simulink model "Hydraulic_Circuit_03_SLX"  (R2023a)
settings: Solver=ode23s  StartTime=0.0  StopTime=10.0  MaxStep=0.001  RelTol=1e-3
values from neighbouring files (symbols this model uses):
  C_5 = 0.001*m^3/Pa    (= 0.001)    [Hydraulic_Circuit_03_EQN.m]    (also in Hydraulic_Circuit_03_SLX_m.m; Electric_Circuit_02_EQN.m; Electric_Circuit_02_SLX_m.m; Electric_Circuit_04_EQN.m)
  C_8 = 0.001*m^3/Pa    (= 0.001)    [Hydraulic_Circuit_03_EQN.m]    (also in Hydraulic_Circuit_03_SLX_m.m; BIG_EC_Simscape_EQN.m; BIG_EC_Simscape_SLX_m.m; Electric_Circuit_11_EQN.m)
  L_4 = 10*Pa*sec^2/m^3    (= 10)    [Hydraulic_Circuit_03_EQN.m]    (also in Hydraulic_Circuit_03_SLX_m.m; Electric_Circuit_02_EQN.m = 0.002; Electric_Circuit_02_SLX_m.m = 0.002; Electric_Circuit_03_EQN.m = 0.002)
  L_6 = 10*Pa*sec^2/m^3    (= 10)    [Hydraulic_Circuit_03_EQN.m]    (also in Hydraulic_Circuit_03_SLX_m.m; Electric_Circuit_07_EQN.m = 0.002; Electric_Circuit_07_SLX_m.m = 0.002; Hydraulic_Circuit_02_EQN.m)
  P_1_0 = 10*Pa    (= 10)    [Hydraulic_Circuit_03_SLX_m.m]    (also in Hydraulic_Circuit_01_SLX_m.m; Hydraulic_Circuit_02_SLX_m.m; Hydraulic_Clutch_System_SLX_m.m)
  P_5_0 = 0*Pa    (= 0)    [Hydraulic_Circuit_03_SLX_m.m]    (also in Hydraulic_Circuit_02_SLX_m.m)
  P_8_0 = 0*Pa    (= 0)    [Hydraulic_Circuit_03_SLX_m.m]
  Q_4_0 = 0*m^3/sec    (= 0)    [Hydraulic_Circuit_03_SLX_m.m]    (also in Hydraulic_Circuit_02_SLX_m.m)
  Q_6_0 = 0*m^3/sec    (= 0)    [Hydraulic_Circuit_03_SLX_m.m]    (also in Hydraulic_Circuit_02_SLX_m.m)
  Q_b_0 = 0*m^3/sec    (= 0)    [Hydraulic_Circuit_03_SLX_m.m]
  R_2 = 10000*Pa/(m^3/sec)    (= 10000)    [Hydraulic_Circuit_03_EQN.m]    (also in Hydraulic_Circuit_03_SLX_m.m; BIG_EC_Simscape_EQN.m = 100; BIG_EC_Simscape_SLX_m.m = 100; Electric_Circuit_07_EQN.m = 100)
  R_3 = 10000*Pa/(m^3/sec)    (= 10000)    [Hydraulic_Circuit_03_EQN.m]    (also in Hydraulic_Circuit_03_SLX_m.m; Electric_Circuit_01_EQN.m = 100; Electric_Circuit_01_SLX_m.m = 100; Electric_Circuit_02_EQN.m = 100)
  R_7 = 10000*Pa/(m^3/sec)    (= 10000)    [Hydraulic_Circuit_03_EQN.m]    (also in Hydraulic_Circuit_03_SLX_m.m; BIG_EC_Simscape_EQN.m = 100; BIG_EC_Simscape_SLX_m.m = 100; Electric_Circuit_03_EQN.m = 100)
  R_9 = 10000*Pa/(m^3/sec)    (= 10000)    [Hydraulic_Circuit_03_EQN.m]    (also in Hydraulic_Circuit_03_SLX_m.m)
  Ts = Tfin/Nr_Ts_Points    (= 0.01999875)    [Hydraulic_Circuit_03_SLX_m.m]    (also in BIG_EC_Simscape_SLX_m.m = 0.0003; Car_Dumper_SLX_m.m = 0.0022779; Electric_Circuit_01_SLX_m.m = 0.005; Electric_Circuit_02_SLX_m.m = 0.000480145)

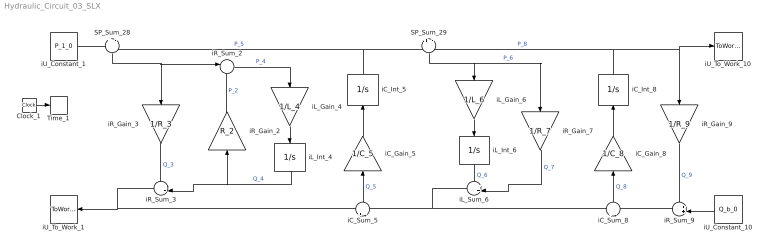
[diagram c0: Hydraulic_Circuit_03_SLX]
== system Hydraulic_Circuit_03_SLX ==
  Clock_1 : Clock
  SP_Sum_28 : Sum  Inputs=+|-
  SP_Sum_29 : Sum  Inputs=+|-
  Time_1 : ToWorkspace  VariableName=t  SaveFormat=Timeseries  SampleTime=Ts
  iC_Gain_5 : Gain  Gain=1/C_5  Multiplication=Matrix(K*u)
  iC_Gain_8 : Gain  Gain=1/C_8  Multiplication=Matrix(K*u)
  iC_Int_5 : Integrator  InitialCondition=P_5_0
  iC_Int_8 : Integrator  InitialCondition=P_8_0
  iC_Sum_5 : Sum  Inputs=+|-
  iC_Sum_8 : Sum  Inputs=+|-
  iL_Gain_4 : Gain  Gain=1/L_4  Multiplication=Matrix(K*u)
  iL_Gain_6 : Gain  Gain=1/L_6  Multiplication=Matrix(K*u)
  iL_Int_4 : Integrator  InitialCondition=Q_4_0
  iL_Int_6 : Integrator  InitialCondition=Q_6_0
  iL_Sum_6 : Sum  Inputs=++|
  iR_Gain_2 : Gain  Gain=R_2  Multiplication=Matrix(K*u)
  iR_Gain_3 : Gain  Gain=1/R_3  Multiplication=Matrix(K*u)
  iR_Gain_7 : Gain  Gain=1/R_7  Multiplication=Matrix(K*u)
  iR_Gain_9 : Gain  Gain=1/R_9  Multiplication=Matrix(K*u)
  iR_Sum_2 : Sum  Inputs=|+-
  iR_Sum_3 : Sum  Inputs=++|
  iR_Sum_9 : Sum  Inputs=++|
  iU_Constant_1 : Constant  Value=P_1_0
  iU_Constant_10 : Constant  Value=Q_b_0
  iU_To_Work_1 : ToWorkspace  VariableName=Q_1_0  SaveFormat=Timeseries  SampleTime=Ts
  iU_To_Work_10 : ToWorkspace  VariableName=P_b_0  SaveFormat=Timeseries  SampleTime=Ts
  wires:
  iU_Constant_1/1 -> SP_Sum_28/1
  iC_Int_5/1 -> SP_Sum_28/2, SP_Sum_29/1  "P_5"
  iR_Sum_3/1 -> iU_To_Work_1/1, iC_Sum_5/1
  SP_Sum_28/1 -> iR_Gain_3/1, iR_Sum_2/1
  iL_Int_4/1 -> iR_Sum_3/2, iR_Gain_2/1  "Q_4"
  iR_Gain_3/1 -> iR_Sum_3/1  "Q_3"
  iR_Sum_2/1 -> iL_Gain_4/1  "P_4"
  iR_Gain_2/1 -> iR_Sum_2/2  "P_2"
  iL_Gain_4/1 -> iL_Int_4/1
  iL_Sum_6/1 -> iC_Sum_5/2, iC_Sum_8/1
  iC_Sum_5/1 -> iC_Gain_5/1  "Q_5"
  iC_Gain_5/1 -> iC_Int_5/1
  iC_Int_8/1 -> SP_Sum_29/2, iU_To_Work_10/1, iR_Gain_9/1  "P_8"
  SP_Sum_29/1 -> iL_Gain_6/1, iR_Gain_7/1  "P_6"
  iR_Gain_7/1 -> iL_Sum_6/2  "Q_7"
  iL_Gain_6/1 -> iL_Int_6/1
  iL_Int_6/1 -> iL_Sum_6/1  "Q_6"
  iR_Sum_9/1 -> iC_Sum_8/2
  iC_Sum_8/1 -> iC_Gain_8/1  "Q_8"
  iC_Gain_8/1 -> iC_Int_8/1
  iU_Constant_10/1 -> iR_Sum_9/2
  iR_Gain_9/1 -> iR_Sum_9/1  "Q_9"
  Clock_1/1 -> Time_1/1
